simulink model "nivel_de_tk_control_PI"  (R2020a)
settings: Solver=ode45  StartTime=0.0  StopTime=15  RelTol=1e-6  EnableMultiTasking=on
libraries: simulink x1

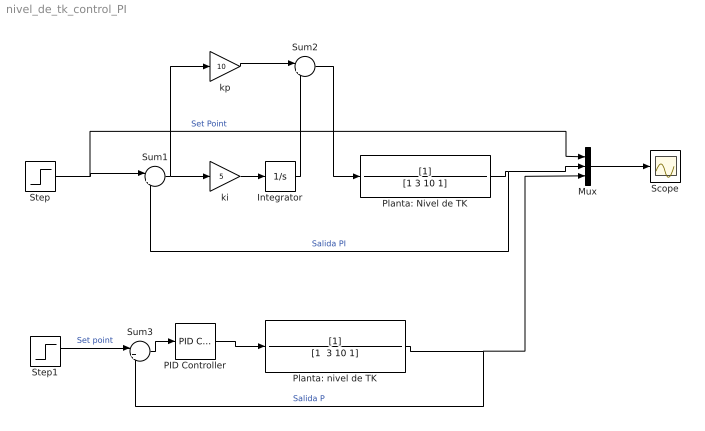
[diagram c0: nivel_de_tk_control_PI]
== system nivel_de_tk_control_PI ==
  Integrator : Integrator
  Mux : Mux  Inputs=3
  PID Controller : simulink/Continuous/PID Controller  Controller=PID  Form=Parallel  TimeDomain=Continuous-time  UseExternalTs=off  SampleTime=-1  IntegratorMethod=Forward Euler  FilterMethod=Forward Euler  ControllerParametersSource=internal  P=17.4  I=17.4  D=4.35  UseFilter=on  N=100  TunerSelectOption=Transfer Function Based (PID Tuner App)  InitialConditionSource=internal  InitialConditionForIntegrator=0  InitialConditionForFilter=0  DifferentiatorICPrevScaledInput=0  ExternalReset=none  TrackingMode=off  Kt=1  LimitOutput=off  UpperSaturationLimit=inf  LowerSaturationLimit=-inf  LinearizeAsGain=on  AntiWindupMode=none  Kb=1  POutMin=[]  POutMax=[]  IOutMin=[]  IOutMax=[]  DOutMin=[]  DOutMax=[]  NOutMin=[]  NOutMax=[]  SumOutMin=[]  SumOutMax=[]  SaturationOutMin=[]  SaturationOutMax=[]  PParamMin=[]  PParamMax=[]  IParamMin=[]  IParamMax=[]  DParamMin=[]  DParamMax=[]  NParamMin=[]  NParamMax=[]  KbParamMin=[]  KbParamMax=[]  KtParamMin=[]  KtParamMax=[]  KbOutMin=[]  KbOutMax=[]  KtOutMin=[]  KtOutMax=[]  IntegratorOutMin=[]  IntegratorOutMax=[]  FilterOutMin=[]  FilterOutMax=[]  SumI1OutMin=[]  SumI1OutMax=[]  SumI2OutMin=[]  SumI2OutMax=[]  SumI3OutMin=[]  SumI3OutMax=[]  SumI4OutMin=[]  SumI4OutMax=[]  SumDOutMin=[]  SumDOutMax=[]  DifferentiatorOutMin=[]  DifferentiatorOutMax=[]  FilterDiffOutCoefMin=[]  FilterDiffOutCoefMax=[]  ReciprocalOutMin=[]  ReciprocalOutMax=[]  SumDenOutMin=[]  SumDenOutMax=[]  SumNumOutMin=[]  SumNumOutMax=[]  DivideOutMin=[]  DivideOutMax=[]  UdiffTsProdOutMin=[]  UdiffTsProdOutMax=[]  NTsProdOutMin=[]  NTsProdOutMax=[]  UintegralTsProdOutMin=[]  UintegralTsProdOutMax=[]  UngainTsProdOutMin=[]  UngainTsProdOutMax=[]  IntegratorContinuousStateAttributes=''  IntegratorStateMustResolveToSignalObject=off  IntegratorRTWStateStorageClass=Auto  FilterContinuousStateAttributes=''  FilterStateMustResolveToSignalObject=off  FilterRTWStateStorageClass=Auto  ParallelPVariant=InternalParameters  IdealPVariant=Disabled  IVariant=InternalParameters  DVariant=InternalParameters  IntegratorVariant=Continuous  SatVariant=Disabled  AWVariant=Passthrough  PCopyVariant=Disabled  TRVariant=Disabled  FdbkBlocksVariant=Forward  IdealPFdbkVariant=Disabled  SatFdbkVariant=Disabled  DerivativeFilterVariant=ContFilter  NVariant=InternalParameters  NCopyVariant=Disabled  FilterICVariant=InternalICsFilter  IntegratorICVariant=InternalICs  ExternalResetVariant=Disabled  TRSumVariant=Passthrough  SumFdbkVariant=Disabled  SumVariant=Sum_PID  TsampFilterVariant=InternalTs  TsampNgainVariant=Passthrough  TsampIntegralVariant=Passthrough
  Planta: Nivel de TK : TransferFcn  Denominator=[1 3 10 1]
  Planta: nivel de TK : TransferFcn  Denominator="[1  3 10 1]"
  Scope : Scope
  Step : Step  Time=0  SampleTime=0
  Step1 : Step  Time=0  SampleTime=0
  Sum1 : Sum  Inputs=|+-
  Sum2 : Sum  Inputs=|++
  Sum3 : Sum  Inputs=|+-
  ki : Gain  Gain=5
  kp : Gain  Gain=10
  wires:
  Step/1 -> Sum1/1, Mux/1  "Set Point"
  Sum1/1 -> ki/1, kp/1
  Planta: Nivel de TK/1 -> Mux/2, Sum1/2  "Salida PI"
  Mux/1 -> Scope/1
  kp/1 -> Sum2/1
  Sum2/1 -> Planta: Nivel de TK/1
  ki/1 -> Integrator/1
  Integrator/1 -> Sum2/2
  Planta: nivel de TK/1 -> Mux/3, Sum3/2  "Salida P"
  Step1/1 -> Sum3/1  "Set point"
  PID Controller/1 -> Planta: nivel de TK/1
  Sum3/1 -> PID Controller/1
